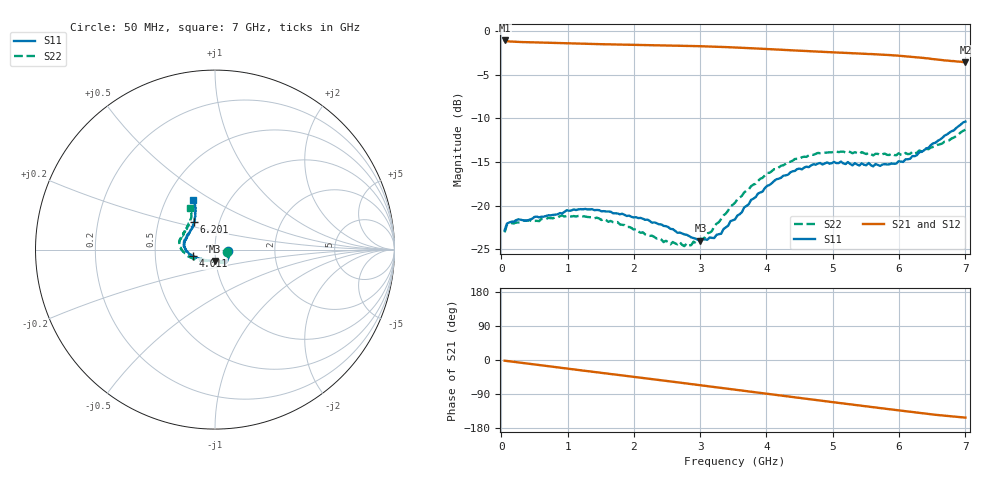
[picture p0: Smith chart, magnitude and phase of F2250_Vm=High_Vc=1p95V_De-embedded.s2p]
! Integrated Device Technology
! Corporate Headquarters
! 6024 Silver Creek Valley Road
! San Jose, CA 95138  USA
! Phone:  1-408-284-8200
! Toll Free:  1-800-223-1366
! Webpage:  http://www.idt.com/
! Timing and RF Division
! 515 Groton Road, Suite 102
! Westford, MA 01886-6024
! Device:  F2250
! Description: Voltage Variable RF Attenuator
! Frequency:  50.0 -  6000.00 MHz
! Package:  3x3 mm Thin QFN Plastic Package: 16 pin
! Ports:  2 RF, 3 DC
!  Pin  1  = GND
!  Pin  2  = NC
!  Pin  3  = RF1  = Port 1
!  Pin  4  = NC
!  Pin  5  = GND
!  Pin  6  = GND
!  Pin  7  = GND
!  Pin  8  = GND
!  Pin  9  = NC
!  Pin 10  = RF2  = Port 2
!  Pin 11  = NC
!  Pin 12  = GND
!  Pin 13  = GND
!  Pin 14  = VCNTRL
!  Pin 15  = VDD
!  Pin 16  = VMODE
! Vcntrl:  1.950 Volts
! Vmode:  +3.300 Volts
! Vdd:  +3.30  Volts
! Current:  1.321 mA
! Data:  The device was measured on a the F2250 evaluation board which has
!  individual transmission lines to the RF pins.  Data was collected
!  using a calibrated network analyzer.  The evaluation board was
!  de-embedded using a TRL calibration technique.
!  The reference plane is the edge of the package pin.
! Misc:  SN 10
!  Action Tracker AT0258
! Date Measured:  2014-11-26
! Date:  2015-10-15  MJV
! Note:
!  Integrated Device Technology supplies this data as a sample of measured
!  data at the package pin for this product.  Your particular data for this
!  product may vary.
!  Data was taken at 25 degrees C.
!  Integrated Device Technology reserves the right to change this data at anytime.
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# GHz S dB R 50
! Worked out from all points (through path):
!   201 points, 50 MHz to 7 GHz, reference 50 ohm
!   highest |S21| = -1.09 dB at 50 MHz (marker M1); lowest = -3.6 dB at 7 GHz (marker M2)
!   group delay of S21, straight-line fit = 61.1 ps
!   lowest |S11| = -24.0 dB at 3.004 GHz (marker M3), VSWR 1.13, Z = 49.8 - j6.3 ohm
!   |S11| at or under -10 dB: start of sweep to end of sweep
!   |S22| runs from -24.6 to -11.3 dB; largest |S21 - S12| = 0.0019
!   S11 on the Smith chart (normalised r, x): 50 MHz: 1.15, -0.02; 4.011 GHz: 0.78, -0.06; 6.201 GHz: 0.76, +0.24; 7 GHz: 0.68, +0.42
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0.05  -22.82 -7.8  -1.09 -1.8  -1.09 -1.8  -23.05 -8.7
0.08475  -22.05 -7.3  -1.17 -2.5  -1.17 -2.5  -22.18 -7.8
0.1195  -21.92 -7.9  -1.20 -3.3  -1.20 -3.3  -22.00 -7.6
0.71025  -21.09 -33.0  -1.35 -16.4  -1.35 -16.4  -21.38 -35.6
1.2315  -20.41 -49.4  -1.46 -27.9  -1.46 -27.9  -21.22 -56.1
1.75275  -20.88 -56.2  -1.56 -39.1  -1.56 -39.1  -21.87 -64.8
2.37825  -22.13 -57.6  -1.64 -52.7  -1.65 -52.7  -23.71 -70.4
2.552  -22.65 -61.6  -1.67 -56.6  -1.67 -56.6  -24.42 -77.0
2.691  -23.08 -67.7  -1.69 -59.7  -1.69 -59.7  -24.15 -83.6
2.7605  -23.29 -69.4  -1.70 -61.2  -1.70 -61.2  -24.63 -87.6
3.00375  -24.01 -88.5  -1.75 -66.7  -1.75 -66.7  -23.78 -107.6
3.21225  -23.70 -109.1  -1.79 -71.4  -1.79 -71.4  -22.35 -125.1
3.525  -21.57 -138.0  -1.89 -78.5  -1.89 -78.5  -19.67 -144.0
3.76825  -19.32 -153.8  -1.98 -84.0  -1.98 -84.0  -17.76 -155.7
4.0115  -17.72 -164.2  -2.07 -89.4  -2.07 -89.4  -16.25 -165.6
4.4285  -16.02 -177.0  -2.24 -98.6  -2.24 -98.6  -14.65 -178.7
4.7065  -15.25 175.5  -2.34 -104.7  -2.34 -104.8  -14.18 175.2
5.054  -15.12 167.1  -2.47 -112.4  -2.46 -112.5  -13.80 167.8
5.85325  -15.27 140.5  -2.76 -129.9  -2.76 -130.0  -14.19 148.6
6.20075  -14.32 127.9  -2.97 -137.6  -2.97 -137.7  -13.83 139.3
6.54825  -12.79 119.0  -3.24 -144.6  -3.24 -144.7  -13.23 127.9
7  -10.37 113.5  -3.57 -152.0  -3.58 -152.1  -11.30 121.4
